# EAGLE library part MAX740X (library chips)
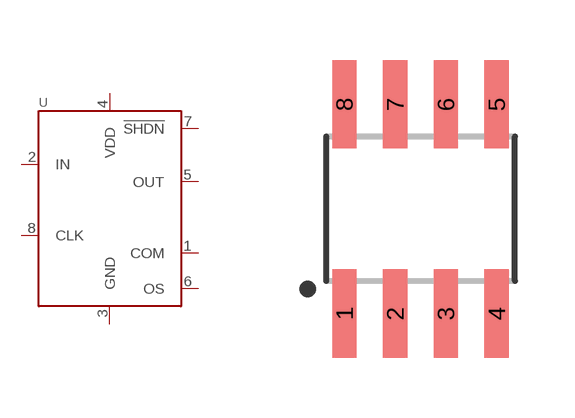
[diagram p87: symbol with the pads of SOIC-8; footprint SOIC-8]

Designator prefix U

## MAX740XESA (ROCHESTER_ELECTRONICS: MAX7405ESA)  [SOIC-8]
1  COM
2  IN
3  GND
4  VDD
5  OUT
6  OS
7  !SHDN
8  CLK

## Footprint SOIC-8 (pad centres in mm)
smd 0.61 x 2.21: 1 -1.905,-2.616; 2 -0.635,-2.616; 3 0.635,-2.616; 4 1.905,-2.616; 5 1.905,2.616; 6 0.635,2.616; 7 -0.635,2.616; 8 -1.905,2.616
